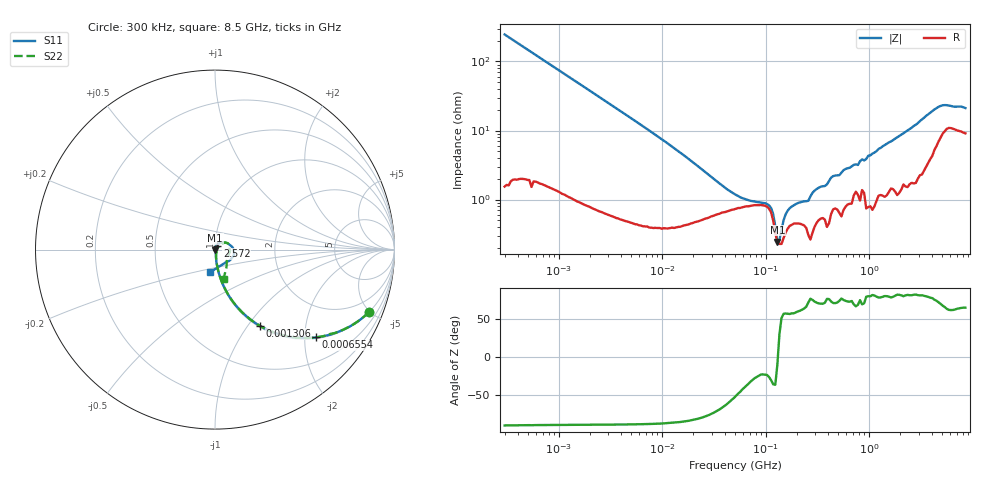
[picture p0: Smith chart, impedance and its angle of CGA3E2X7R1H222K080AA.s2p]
! S-parameter Generated by TDK Corporation
! Copyright(C) 2015 TDK Corporation.
! All Rights Reserved.
! TDK P/N: CGA3E2X7R1H222K080AA (Multilayer Ceramic Chip Capacitors)
! Property: C=2.2nF
! Size(LxWxT): 1.6x0.8x0.8mm, 0.063x0.031x0.031inches
! Model Type: s2p (Touchstone File Format Version 1.0)
! Frequency: DC=Yes Start=0.3MHz Stop=8500MHz 225points Log-sweep
! Note:
! Model Generated on Jun. 23, 2015
! Hash(MD5):
! Port Assignments:
!  1 ---| |--- 2
! Applicable Conditions:
!  Temperature = 25 degC
!  DC Bias Voltage = 0 V
!  Small Signal Operation
! Terms and conditions regarding TDK Simulation Models
! (1)This simulation model is being provided solely for informational purposes. Please refer to the specifications of the products in terms of detailed characteristics of such products.
! (2)In no event shall TDK Corporation of any of its subsidiaries be liable for any loss or damage arising, directly or indirectly,
!  From any information contained in this simulation model, including, but not limited to loss or damages arising from any inaccuracies, omissions or errors in connection with such information.
! (3)Any and all copyrights on this simulation model are owned by TDK Corporation.
!  Duplication or redistribution of this simulation model without prior written permission from TDK Corporation is prohibited.
! (4)This simulation model is subject to any modification or change without any prior notice.
! (5)Neither TDK Corporation nor any of its subsidiaries shall make any warranty, express or implied,
!  Including but not limited to the correctness, implied warranties of merchantability and fitness for a particular purpose with respect to this simulation models.
! (6)The use of this simulation model shall be deemed to have consented to the terms and conditions hereof.
# MHz S MA R 50
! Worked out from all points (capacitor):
!   224 points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, 300 kHz to 8.5 GHz, reference 50 ohm
!   read as one part in series: C = 2.15 nF near 314.1 kHz
!   lowest |Z| = 242 mohm at 129.6 MHz (marker M1)
!   series resonance near 131.1 MHz, so ESL is about 690 pH
!   S11 on the Smith chart (normalised r, x): 300 kHz: 1.01, -4.90; 655.4 kHz: 1.03, -2.27; 1.306 MHz: 1.02, -1.15; 2.572 GHz: 1.03, +0.04; 8.5 GHz: 0.92, -0.24
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0.3  0.9254 -22.2  0.3761 67.5  0.3758 67.9  0.9256 -22.1
0.6554417  0.7455 -41.0  0.6562 48.2  0.6543 48.4  0.7454 -41.0
1.306219  0.4951 -59.3  0.862 29.6  0.8594 29.8  0.4949 -59.4
1.72111  0.3985 -65.5  0.9114 23.4  0.9088 23.6  0.3982 -65.5
9.430415  0.0788 -83.1  0.9943 4.3  0.9919 4.6  0.07849 -82.8
51.67171  0.01017 -65.4  0.9932 0.2  0.9909 0.5  0.01659 -55.7
129.5872  0.004478 -74.0  0.9968 -0.4  0.9945 -0.1  0.006345 -93.6
246.6485  0.004233 174.2  0.9901 -1.3  0.9879 -1.0  0.006729 -111.8
283.1228  0.005276 -159.7  0.9911 -1.6  0.9889 -1.3  0.001828 162.3
408.9767  0.003375 -104.4  0.9899 -2.1  0.9877 -1.9  0.006482 120.0
514.6664  0.0003117 9.7  0.9866 -2.5  0.9843 -2.2  0.005237 131.2
538.8791  0.001451 -114.6  0.9883 -2.7  0.9858 -2.4  0.00824 104.4
618.5683  0.0008002 -120.6  0.9842 -3.0  0.9821 -2.7  0.008459 82.4
853.3868  0.01154 27.3  0.9843 -3.9  0.9825 -3.7  0.01226 15.6
979.5854  0.008463 79.6  0.9891 -4.7  0.9867 -4.4  0.007042 20.4
1025.67  0.008945 85.2  0.9849 -4.8  0.9823 -4.5  0.0007194 130.1
1073.923  0.006836 61.5  0.9877 -4.9  0.9852 -4.6  0.01092 90.5
1124.446  0.001851 78.6  0.9861 -5.4  0.9838 -5.1  0.006491 66.2
1232.735  0.009332 27.9  0.9845 -5.7  0.9825 -5.4  0.01347 62.5
1551.304  0.012 40.5  0.9811 -7.1  0.979 -6.8  0.01353 65.1
2572.272  0.02461 57.0  0.9769 -11.3  0.9743 -11.2  0.02275 44.9
8500  0.1292 -102.5  0.8891 -31.6  0.8877 -30.7  0.1693 -73.7
